(* Logix 5000 AddOnInstructionDefinition export MRSE_Yaskawa; software revision 17.00 *)

TYPE Yaskawa_EIP_Servo :   // Yaskawa SigmaLogic Axis Structure v2.4.0
STRUCT
   O : Yaskawa_OUT_to_Servo;
   I : Yaskawa_IN_from_Servo;
   AOI_SB : Yaskawa_AOI_Status_Bits;
END_STRUCT
END_TYPE

TYPE Yaskawa_OUT_to_Servo :   // Structure of data sent out to the Yaskawa SigmaLogic controller v2.4.0
STRUCT
   b00_ServoOn : BOOL;   // Servo On
   b01_Stop : BOOL;   // Stops All Current Motion in Progress
   b02_Home : BOOL;   // Start Homing Process
   b03_MoveStart1 : BOOL;   // Start Current Motion
   b06_SuperImpose : BOOL;
   b07_ServoAlarmReset : BOOL;   // Servo Alarm Reset
   b08_ControllerAlarmReset : BOOL;   // SigmaLogic Alarm Reset
   b09_MoveStart2 : BOOL;   // Start Second Motion (Blended Move)
   b10_MoveAbort : BOOL;   // Abort Current Move
   b11_MovePause : BOOL;   // Pause Current Move
   b12_SeqPause : BOOL;   // Indexing Sequence Pause
   b13_SeqResume : BOOL;   // Indexing Sequence Resume
   b14_SeqCancel : BOOL;   // Indexing Sequence Cancel
   b15_AbsEncoderReset : BOOL;   // Absolute Encoder Reset
   b16_SeqStart : BOOL;   // Start Indexing Sequence
   b17_SeqEditSpeed : BOOL;   // Enter Edit Speed
   b18_SeqEditDistance : BOOL;   // Enter Distance Edit
   b19_PLSEnable : BOOL;   // Enable PLS execution
   b20_PLSActivateOutput1 : BOOL;   // Activate PLS output1 switch logic
   b21_PLSActivateOutput2 : BOOL;   // Activate PLS output2 switch logic
   b22_PLSActivateOutput3 : BOOL;   // Activate PLS output3 switch logic
   b23_PLSActivateOutput4 : BOOL;   // Activate PLS output4 switch logic
   b24_SetClock : BOOL;   // Set the remote controller clock with data provided by the PLC
   RebootController : BOOL;
   UseExternalEncoder : BOOL;   // Use External Encoder when executing MAHSP_Yaskawa
   b32_HeatbeatAnswer : BOOL;   // Heartbeat Answer
   BrakeBypassRequest : BOOL;
   SetFwdTorqueLimit : BOOL;
   SetRevTorqueLimit : BOOL;
   TorqueLimit : DINT;
   TorqueRamp : DINT;
   HomeMethod : INT;
   HomeSpeed : DINT;
   HomeAccDec : DINT;   // Home Move Acceleration/Deceleration Rate
   HomeBackOffDistance : DINT;
   HomeCreepSpeed : DINT;
   HomeCreepDistanceLimit : DINT;
   HomeCreepTimeLimit : DINT;
   HomeOffsetDistance : DINT;
   HomeOffsetSpeed : DINT;
   HomePostion : DINT;
   HomeTorque : DINT;
   HomeInputNo : DINT;
   HomeApproachTimeLimit : DINT;
   HomeApproachDistLimit : DINT;
   HomeDirection : INT;
   HomeSwitchMode : INT;
   MoveType : INT;
   MoveDirection : INT;
   MoveAccel1 : DINT;
   MoveAccel2 : DINT;
   MoveDecel1 : DINT;
   MoveDecel2 : DINT;
   MoveSpeed1 : DINT;
   MoveSpeed2 : DINT;
   MoveDistance1 : DINT;
   MoveDistance2 : DINT;
   MovePosition1 : DINT;
   MovePosition2 : DINT;
   RegistrationDistance : DINT;
   GearNumerator : DINT;
   GearDenominator : DINT;
   SuperImposeDistance : DINT;
   Resolution : INT;
   RegistrationDirection : INT;
   TuningLevel : INT;
   SequenceStep : INT;   // Staring Sequence Step Number
   SequenceEditStep : INT;   // Sequence Step Number to Edit
   FlagCommandBits1 : DINT;   // Flag Commands. 1..64 are General Flags, Bits 0..31 correspond to Flag 1..32
   FlagCommandBits2 : DINT;   // Flag Commands cont. 1..64 are General Flags, Bits 0..31 correspond to Flag 33..64
   DigitalOutCommandBits : DINT;   // Digital Output commands. Bits 0-7 correspond to CN13 Digital Outputs 0-7, used as Flag 73-80. Bits 8-10 correspond to CN1 Digital Outputs 0-2 used as Flag 88-90"
   SequenceEditSpeed : DINT;
   SequenceEditDistance : DINT;
   FeedRateOverride : INT;
   HSI_Enable : BOOL;
   HSI_MoveMode : BOOL;   // 0=Relative; 1=Moves per Cycle
   HSI_CalcMethod : BOOL;   // 0=Accel/Decel; 1=Time
   HSI_MoveDirection : BOOL;   // 0 = Negative; 1 = Positive
   HSI_TriggerFlag : INT;
   HSI_MovingFlag : INT;
   HSI_DwellingFlag : INT;
   HSI_DoneFlag : INT;
   HSI_MoveType : INT;   // 0=Single; 1=Repeat; 2=Repeat "x" times
   HSI_RepeatNumber : INT;
   HSI_Distance : DINT;
   HSI_Speed : DINT;
   HSI_Accel : DINT;
   HSI_MoveTime : DINT;
   HSI_DwellTime : DINT;
   PLS_OutputFlag1 : INT;
   PLS_OutputFlag2 : INT;
   PLS_OutputFlag3 : INT;
   PLS_OutputFlag4 : INT;
   PLS_OnPosition1 : DINT;
   PLS_OffPosition1 : DINT;
   PLS_OnPosition2 : DINT;
   PLS_OffPosition2 : DINT;
   PLS_OnPosition3 : DINT;
   PLS_OffPosition3 : DINT;
   PLS_OnPosition4 : DINT;
   PLS_OffPosition4 : DINT;
   PLS_OnCompensation1 : INT;
   PLS_OffCompensation1 : INT;
   PLS_OnCompensation2 : INT;
   PLS_OffCompensation2 : INT;
   PLS_OnCompensation3 : INT;
   PLS_OffCompensation3 : INT;
   PLS_OnCompensation4 : INT;
   PLS_OffCompensation4 : INT;
   RTC_Year : INT;
   RTC_Month : INT;
   RTC_Day : INT;
   RTC_Hour : INT;
   RTC_Min : INT;
   RTC_Sec : INT;
   StopDecel : DINT;
   AnalogOutput : INT;   // CN13, AO_01 [mV]
END_STRUCT
END_TYPE

TYPE Yaskawa_AOI_Status_Bits :   // Internal bits used to interlock Yaskawa AOI execution. v2.4.0
STRUCT
   MAM : BOOL;   // Move AOI Active
   MAJ : BOOL;   // Jog AOI Active
   MAB : BOOL;   // Blending AOI Active
   MAG : BOOL;   // Gearing AOI Active
   MAHSP : BOOL;   // Home SetPoint AOI Active
   MAH : BOOL;   // Homing AOI Active
   MSQE : BOOL;   // Sequence Edit AOI Active
   MSQR : BOOL;   // Sequence Run AOI Active
   MHSI : BOOL;   // High Speed Index AOI Active
   MSO : BOOL;   // Servo On
   MSF : BOOL;   // Servo Off
   MAFR : BOOL;   // Fault Reset
   MAS : BOOL;   // Servo Abort
   MTRQ : BOOL;   // Torque Mode Active
   MPLS : BOOL;   // PLS Active
   MCLK : BOOL;   // SetClock Active
   MSTL : BOOL;   // Set Torque Limit Active
   AOI_Permissive : BOOL;   // Permissive to Execute an AOI
END_STRUCT
END_TYPE

TYPE Yaskawa_IN_from_Servo :   // Structure of data coming from the Yaskawa SigmaLogic controller. v2.4.0
STRUCT
   AlarmText : STRING;   // ServoPack Alarm Code plus Text Description
   b00_Heartbeat : BOOL;
   b01_Alarm : BOOL;   // ServoPack Alarm
   b02_Warning : BOOL;   // ServoPack Warning
   b03_Ready : BOOL;   // ServoPack Ready
   b04_Enabled : BOOL;   // ServoPack Enabled ("Servo On")
   b05_StopComplete : BOOL;
   b06_HomeComplete : BOOL;
   b07_HomeBusy : BOOL;
   b08_HomeActive : BOOL;
   b09_HomeAborted : BOOL;
   b10_HomeError : BOOL;
   b11_MoveAbsComplete : BOOL;
   b12_MoveAbsBusy : BOOL;
   b13_MoveAbsActive : BOOL;
   b14_MoveAbsAborted : BOOL;
   b15_MoveAbsError : BOOL;
   b16_MoveRelComplete : BOOL;
   b17_MoveRelBusy : BOOL;
   b18_MoveRelActive : BOOL;
   b19_MoveRelAborted : BOOL;
   b20_MoveRelError : BOOL;
   b21_JogAtSpeed : BOOL;
   b22_JogBusy : BOOL;
   b23_JogActive : BOOL;
   b24_JogAborted : BOOL;
   b25_JogError : BOOL;
   b26_GearInSync : BOOL;
   b27_GearBusy : BOOL;
   b28_GearActive : BOOL;
   b29_GearAborted : BOOL;
   b30_GearError : BOOL;
   b32_MoveSuperComplete : BOOL;
   b33_MoveSuperBusy : BOOL;
   b34_MoveSuperActive : BOOL;
   b35_MoveSuperAborted : BOOL;
   b36_MoveSuperError : BOOL;
   b37_PowerCycleRequired : BOOL;
   b38_MoveBlend1Complete : BOOL;
   b39_MoveBlend1Busy : BOOL;
   b40_MoveBlend1Active : BOOL;
   b41_MoveBlend1Abort : BOOL;
   b42_MoveBlend1Error : BOOL;
   b43_MoveBlend2Complete : BOOL;
   b44_MoveBlend2Busy : BOOL;
   b45_MoveBlend2Active : BOOL;
   b46_MoveBlend2Abort : BOOL;
   b47_MoveBlend2Error : BOOL;
   b48_RegComplete : BOOL;
   b49_RegBusy : BOOL;
   b50_RegActive : BOOL;
   b51_RegAborted : BOOL;
   b52_RegError : BOOL;
   b53_ResetAbsEncoderActive : BOOL;
   b54_ResetAbsEncoderBusy : BOOL;
   b55_ResetAbsEncoderDone : BOOL;
   b56_ResetAbsEncoderError : BOOL;
   b57_SeqRunning : BOOL;
   b58_RegSensorNotReached : BOOL;
   b59_SeqEditError : BOOL;
   b60_SeqEditDone : BOOL;
   b61_TorqueAtTorque : BOOL;
   b62_TorqueBusy : BOOL;
   b63_TorqueActive : BOOL;
   b64_TorqueAborted : BOOL;
   b65_TorqueError : BOOL;
   b66_ControllerAlarm : BOOL;
   b67_ApplicationError : BOOL;
   b68_AxisAtStandStill : BOOL;
   b69_TestModeActive : BOOL;
   b70_ServoParamsOK : BOOL;
   b71_SetFwdTorqueLimitDone : BOOL;
   b72_SetRevTorqueLimitDone : BOOL;
   Position : DINT;
   Speed : DINT;
   Torque : DINT;
   HomeErrorID : INT;
   MoveAbsErrorID : INT;
   MoveRelErrorID : INT;
   JogErrorID : INT;
   GearErrorID : INT;
   MoveSuperErrorID : INT;
   ServoAlarmID : INT;
   ServoWarningID : INT;
   ControllerAlarmID : DINT;
   AxisGenAlarmID : DINT;
   MoveBlend1ErrorID : INT;
   MoveBlend2ErrorID : INT;
   ResetAbsEncoderErrorID : INT;
   FunctionBlockErrorID : INT;
   TorqueErrorID : INT;
   RegErrorID : INT;
   SeqCurrentStep : INT;
   FlagStatusBit1 : DINT;   // Flag Status. 1..64 are General Flags, Bits 0..31 correspond to Flag 1..32
   FlagStatusBit2 : DINT;   // Flag Status cont. 1..64 are General Flags, Bits 0..31 correspond to Flag 33..64
   IOStatusBits : DINT;   // Digital IO Status. Bits 0-7, CN13 Inputs 0-7, Used as Flag 65-72. Bits 8-15, CN13 Outputs 0-7, Used as Flag 73-80. Bits 16-22, CN1 Inputs 0-6, Used as Flag 81-87. Bits 23-25, CN1 Outputs 0-4, Used as Flag 88-92.
   HSI_Moving : BOOL;
   HSI_Dwelling : BOOL;
   HSI_Done : BOOL;
   HSI_Busy : BOOL;
   HSI_Error : BOOL;
   HSI_ErrorCode : INT;
   PLS_Running : BOOL;
   PLS_SwitchStatus1 : BOOL;
   PLS_SwitchStatus2 : BOOL;
   PLS_SwitchStatus3 : BOOL;
   PLS_SwitchStatus4 : BOOL;
   PLS_Busy : BOOL;
   PLS_Error : BOOL;
   PLS_ErrorCode : INT;
   SetClock_Done : BOOL;
   SetClock_Busy : BOOL;
   SetClock_Error : BOOL;
   SetClock_ErrorID : INT;
   SoftwareVersion : DINT;
   FirmwareVersion : DINT;
   CommandedPos : DINT;
   CommandedPosNonCyc : DINT;
   CommandedSpeed : DINT;
   Clock_Year : INT;
   Clock_Month : INT;
   Clock_Day : INT;
   Clock_Hour : INT;
   Clock_Minute : INT;
   Clock_Second : INT;
   AnalogInput : REAL;   // CN13, AI_01 [v]
   BrakeBypassActive : BOOL;
   ForwardTorqueLimit : DINT;
   ReverseTorqueLimit : DINT;
END_STRUCT
END_TYPE

ADD_ON_INSTRUCTION MRSE_Yaskawa   (* revision 2.4 0, ExecuteEnableInFalse *)
// Motion Report Servo Error
// Alarm text will be reported to controller tag at "AxisRef.I.AlarmText"
// Revision note:
// 2.4.0: No functional change
// 2.3.1: No functional change
// 2.3.0: No functional change
// 2.0.0: First release
VAR_INPUT
   AOI_ON_LOCAL : BOOL;
END_VAR
VAR_IN_OUT
   Axis_IN : AB:ETHERNET_MODULE_DINT_256Bytes:I:0; {required}
   Axis : Yaskawa_EIP_Servo; {required}
END_VAR
VAR_OUTPUT
   EN : BOOL; {visible}   // Function is executing
   DN : BOOL; {visible}   // MRSE completed successfully
END_VAR
VAR
   OS1 : BOOL;
   OS2 : BOOL;
END_VAR

ROUTINE EnableInFalse   (* ladder *)
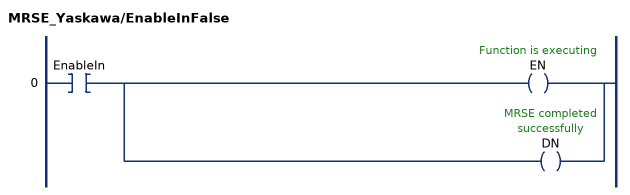
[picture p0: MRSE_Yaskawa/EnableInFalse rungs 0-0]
   0: XIC(EnableIn)[OTE(EN) ,OTE(DN) ];
END_ROUTINE

ROUTINE Logic   (* ladder *)
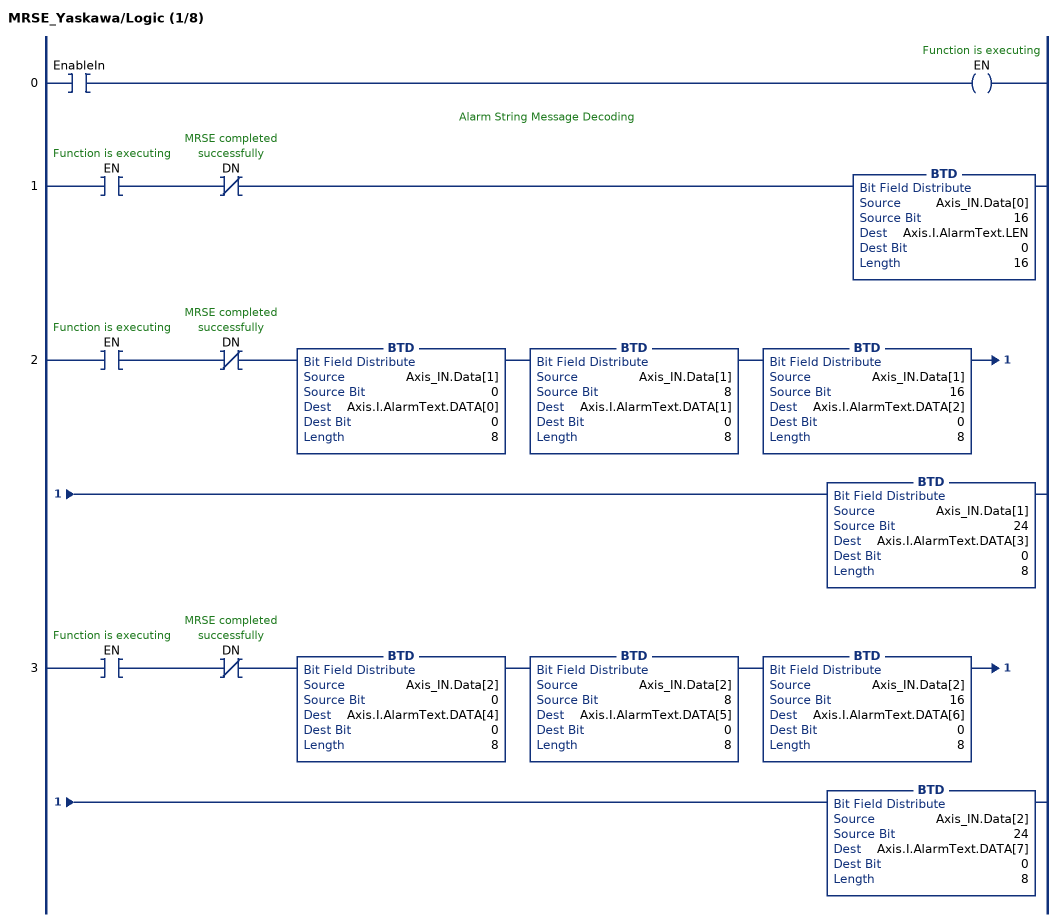
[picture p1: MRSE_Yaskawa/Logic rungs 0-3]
   0: XIC(EnableIn)OTE(EN);
   // Alarm String Message Decoding
   1: XIC(EN)XIO(DN)BTD(Axis_IN.Data[0],16,Axis.I.AlarmText.LEN,0,16);
   2: XIC(EN)XIO(DN)BTD(Axis_IN.Data[1],0,Axis.I.AlarmText.DATA[0],0,8)BTD(Axis_IN.Data[1],8,Axis.I.AlarmText.DATA[1],0,8)BTD(Axis_IN.Data[1],16,Axis.I.AlarmText.DATA[2],0,8)BTD(Axis_IN.Data[1],24,Axis.I.AlarmText.DATA[3],0,8);
   3: XIC(EN)XIO(DN)BTD(Axis_IN.Data[2],0,Axis.I.AlarmText.DATA[4],0,8)BTD(Axis_IN.Data[2],8,Axis.I.AlarmText.DATA[5],0,8)BTD(Axis_IN.Data[2],16,Axis.I.AlarmText.DATA[6],0,8)BTD(Axis_IN.Data[2],24,Axis.I.AlarmText.DATA[7],0,8);
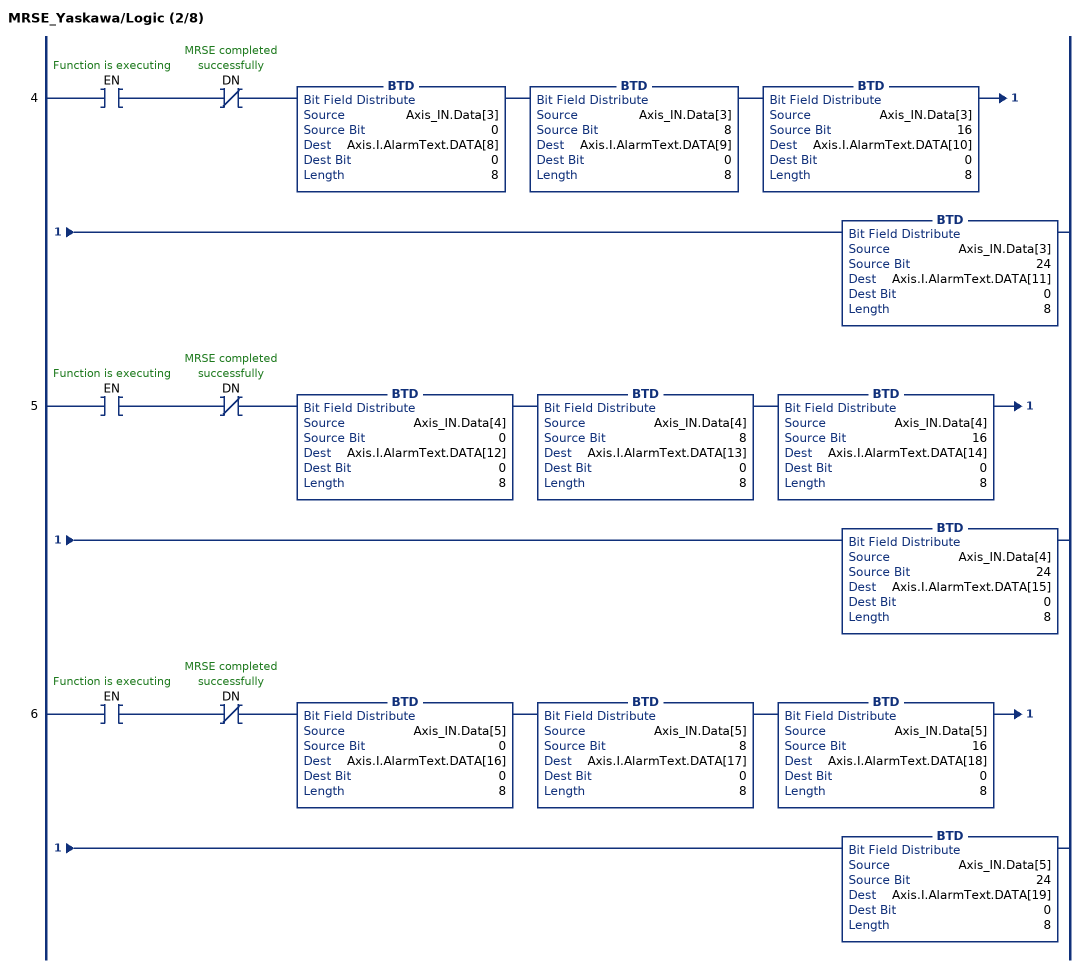
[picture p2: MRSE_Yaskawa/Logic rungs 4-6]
   4: XIC(EN)XIO(DN)BTD(Axis_IN.Data[3],0,Axis.I.AlarmText.DATA[8],0,8)BTD(Axis_IN.Data[3],8,Axis.I.AlarmText.DATA[9],0,8)BTD(Axis_IN.Data[3],16,Axis.I.AlarmText.DATA[10],0,8)BTD(Axis_IN.Data[3],24,Axis.I.AlarmText.DATA[11],0,8);
   5: XIC(EN)XIO(DN)BTD(Axis_IN.Data[4],0,Axis.I.AlarmText.DATA[12],0,8)BTD(Axis_IN.Data[4],8,Axis.I.AlarmText.DATA[13],0,8)BTD(Axis_IN.Data[4],16,Axis.I.AlarmText.DATA[14],0,8)BTD(Axis_IN.Data[4],24,Axis.I.AlarmText.DATA[15],0,8);
   6: XIC(EN)XIO(DN)BTD(Axis_IN.Data[5],0,Axis.I.AlarmText.DATA[16],0,8)BTD(Axis_IN.Data[5],8,Axis.I.AlarmText.DATA[17],0,8)BTD(Axis_IN.Data[5],16,Axis.I.AlarmText.DATA[18],0,8)BTD(Axis_IN.Data[5],24,Axis.I.AlarmText.DATA[19],0,8);
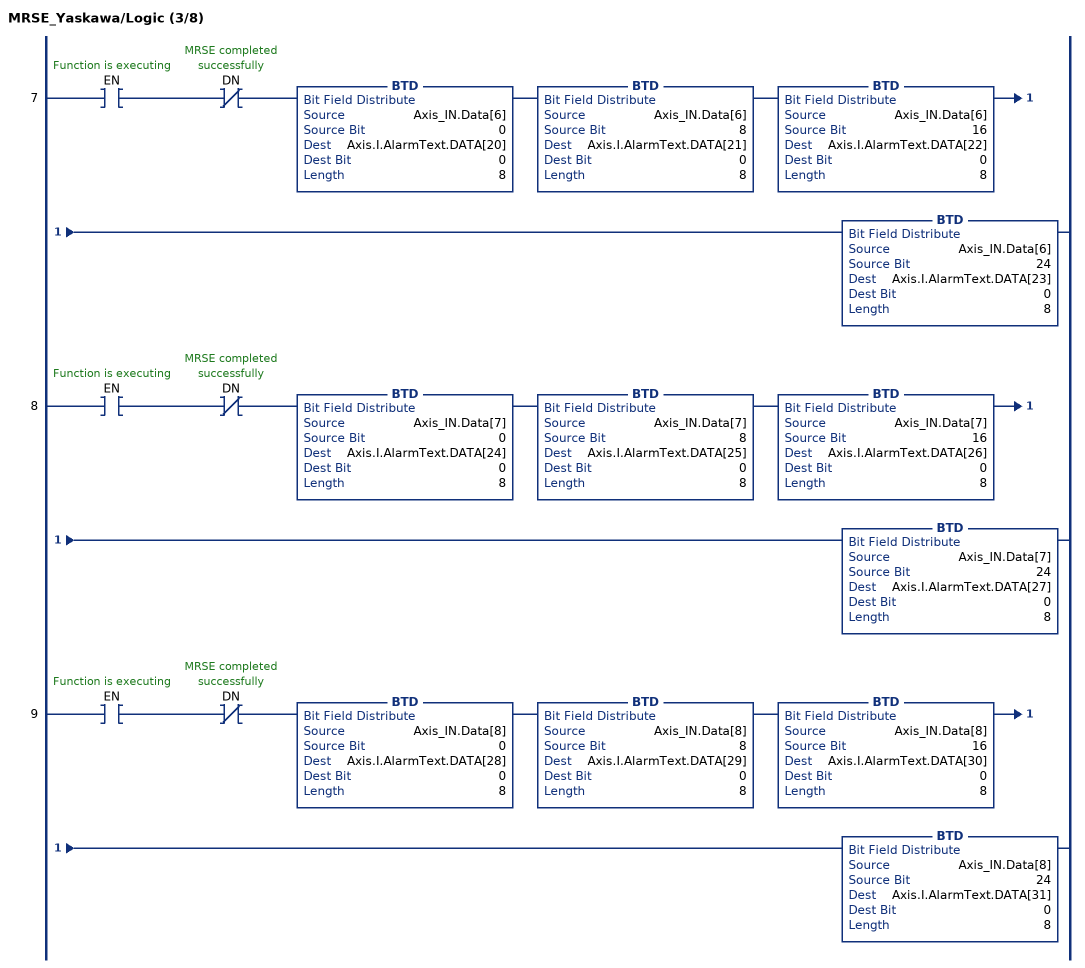
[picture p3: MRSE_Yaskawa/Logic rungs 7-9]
   7: XIC(EN)XIO(DN)BTD(Axis_IN.Data[6],0,Axis.I.AlarmText.DATA[20],0,8)BTD(Axis_IN.Data[6],8,Axis.I.AlarmText.DATA[21],0,8)BTD(Axis_IN.Data[6],16,Axis.I.AlarmText.DATA[22],0,8)BTD(Axis_IN.Data[6],24,Axis.I.AlarmText.DATA[23],0,8);
   8: XIC(EN)XIO(DN)BTD(Axis_IN.Data[7],0,Axis.I.AlarmText.DATA[24],0,8)BTD(Axis_IN.Data[7],8,Axis.I.AlarmText.DATA[25],0,8)BTD(Axis_IN.Data[7],16,Axis.I.AlarmText.DATA[26],0,8)BTD(Axis_IN.Data[7],24,Axis.I.AlarmText.DATA[27],0,8);
   9: XIC(EN)XIO(DN)BTD(Axis_IN.Data[8],0,Axis.I.AlarmText.DATA[28],0,8)BTD(Axis_IN.Data[8],8,Axis.I.AlarmText.DATA[29],0,8)BTD(Axis_IN.Data[8],16,Axis.I.AlarmText.DATA[30],0,8)BTD(Axis_IN.Data[8],24,Axis.I.AlarmText.DATA[31],0,8);
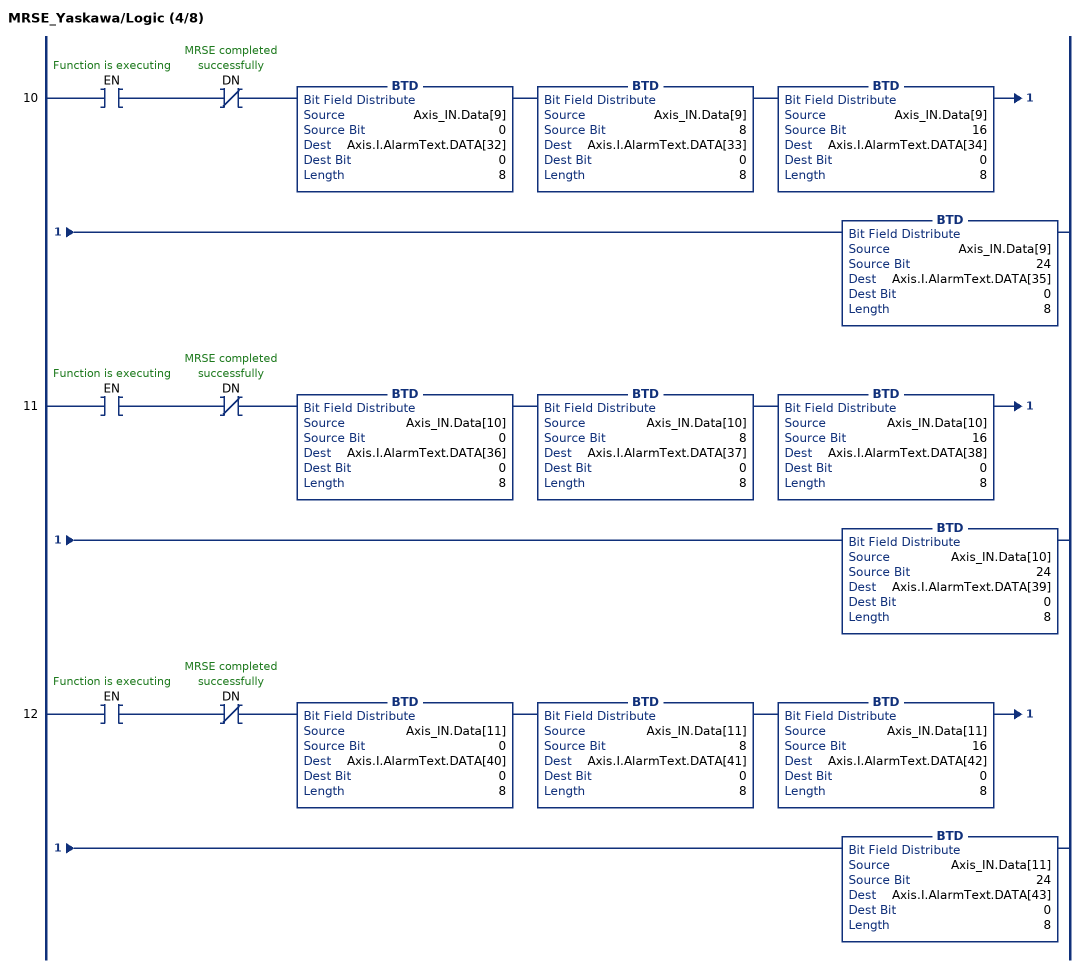
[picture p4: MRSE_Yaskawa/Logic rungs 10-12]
   10: XIC(EN)XIO(DN)BTD(Axis_IN.Data[9],0,Axis.I.AlarmText.DATA[32],0,8)BTD(Axis_IN.Data[9],8,Axis.I.AlarmText.DATA[33],0,8)BTD(Axis_IN.Data[9],16,Axis.I.AlarmText.DATA[34],0,8)BTD(Axis_IN.Data[9],24,Axis.I.AlarmText.DATA[35],0,8);
   11: XIC(EN)XIO(DN)BTD(Axis_IN.Data[10],0,Axis.I.AlarmText.DATA[36],0,8)BTD(Axis_IN.Data[10],8,Axis.I.AlarmText.DATA[37],0,8)BTD(Axis_IN.Data[10],16,Axis.I.AlarmText.DATA[38],0,8)BTD(Axis_IN.Data[10],24,Axis.I.AlarmText.DATA[39],0,8);
   12: XIC(EN)XIO(DN)BTD(Axis_IN.Data[11],0,Axis.I.AlarmText.DATA[40],0,8)BTD(Axis_IN.Data[11],8,Axis.I.AlarmText.DATA[41],0,8)BTD(Axis_IN.Data[11],16,Axis.I.AlarmText.DATA[42],0,8)BTD(Axis_IN.Data[11],24,Axis.I.AlarmText.DATA[43],0,8);
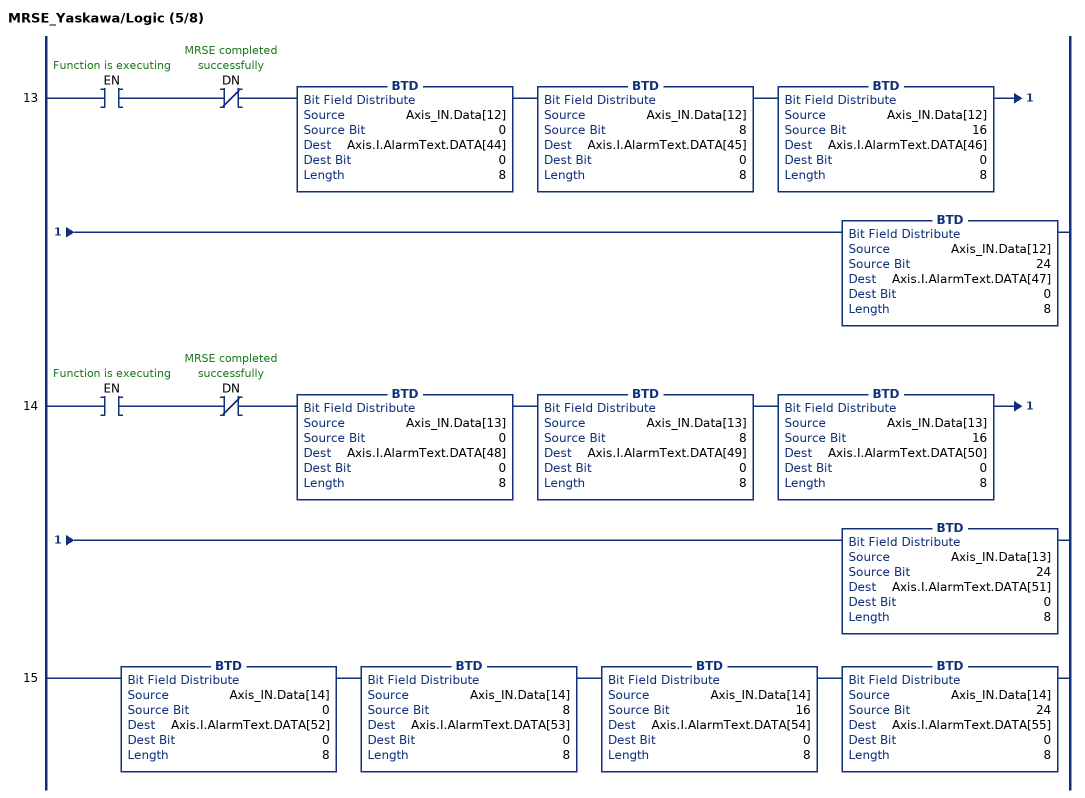
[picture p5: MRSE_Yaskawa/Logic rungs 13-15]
   13: XIC(EN)XIO(DN)BTD(Axis_IN.Data[12],0,Axis.I.AlarmText.DATA[44],0,8)BTD(Axis_IN.Data[12],8,Axis.I.AlarmText.DATA[45],0,8)BTD(Axis_IN.Data[12],16,Axis.I.AlarmText.DATA[46],0,8)BTD(Axis_IN.Data[12],24,Axis.I.AlarmText.DATA[47],0,8);
   14: XIC(EN)XIO(DN)BTD(Axis_IN.Data[13],0,Axis.I.AlarmText.DATA[48],0,8)BTD(Axis_IN.Data[13],8,Axis.I.AlarmText.DATA[49],0,8)BTD(Axis_IN.Data[13],16,Axis.I.AlarmText.DATA[50],0,8)BTD(Axis_IN.Data[13],24,Axis.I.AlarmText.DATA[51],0,8);
   15: BTD(Axis_IN.Data[14],0,Axis.I.AlarmText.DATA[52],0,8)BTD(Axis_IN.Data[14],8,Axis.I.AlarmText.DATA[53],0,8)BTD(Axis_IN.Data[14],16,Axis.I.AlarmText.DATA[54],0,8)BTD(Axis_IN.Data[14],24,Axis.I.AlarmText.DATA[55],0,8);
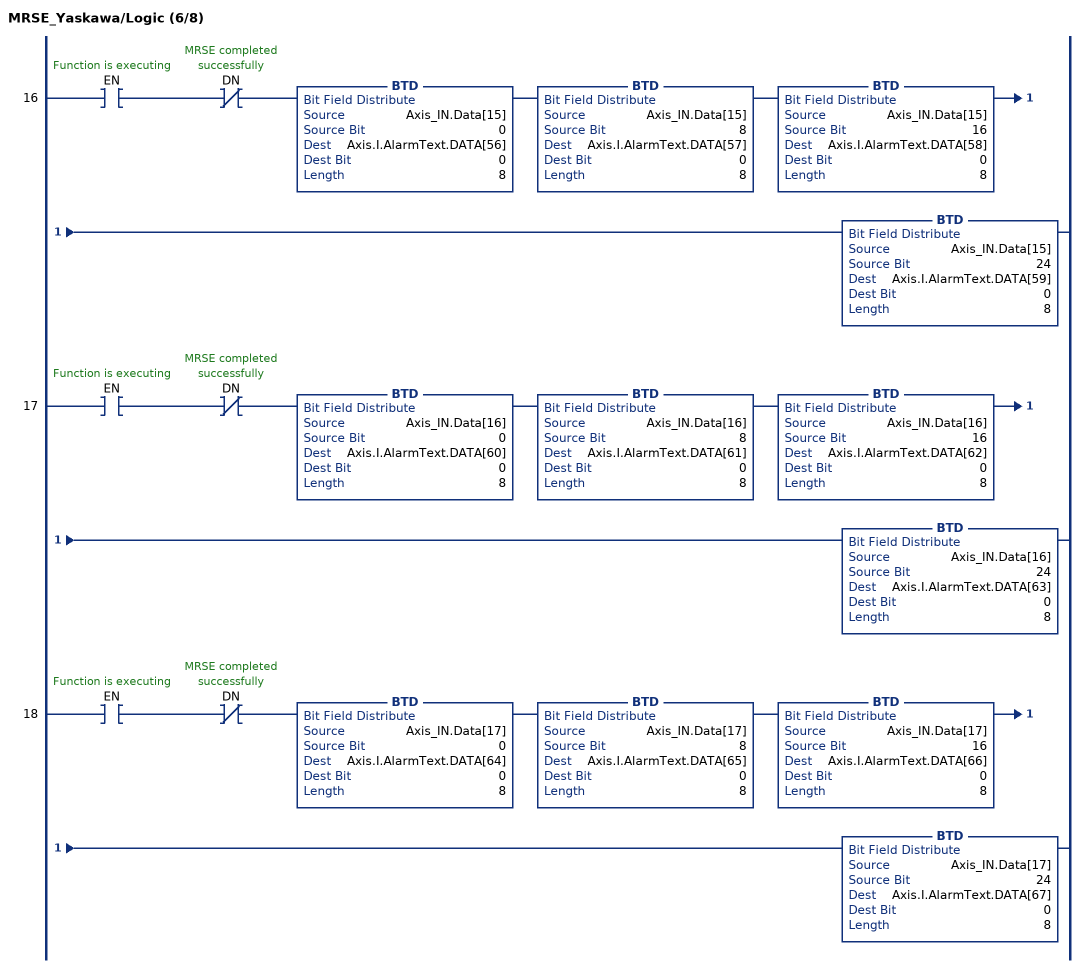
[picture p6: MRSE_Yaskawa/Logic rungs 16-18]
   16: XIC(EN)XIO(DN)BTD(Axis_IN.Data[15],0,Axis.I.AlarmText.DATA[56],0,8)BTD(Axis_IN.Data[15],8,Axis.I.AlarmText.DATA[57],0,8)BTD(Axis_IN.Data[15],16,Axis.I.AlarmText.DATA[58],0,8)BTD(Axis_IN.Data[15],24,Axis.I.AlarmText.DATA[59],0,8);
   17: XIC(EN)XIO(DN)BTD(Axis_IN.Data[16],0,Axis.I.AlarmText.DATA[60],0,8)BTD(Axis_IN.Data[16],8,Axis.I.AlarmText.DATA[61],0,8)BTD(Axis_IN.Data[16],16,Axis.I.AlarmText.DATA[62],0,8)BTD(Axis_IN.Data[16],24,Axis.I.AlarmText.DATA[63],0,8);
   18: XIC(EN)XIO(DN)BTD(Axis_IN.Data[17],0,Axis.I.AlarmText.DATA[64],0,8)BTD(Axis_IN.Data[17],8,Axis.I.AlarmText.DATA[65],0,8)BTD(Axis_IN.Data[17],16,Axis.I.AlarmText.DATA[66],0,8)BTD(Axis_IN.Data[17],24,Axis.I.AlarmText.DATA[67],0,8);
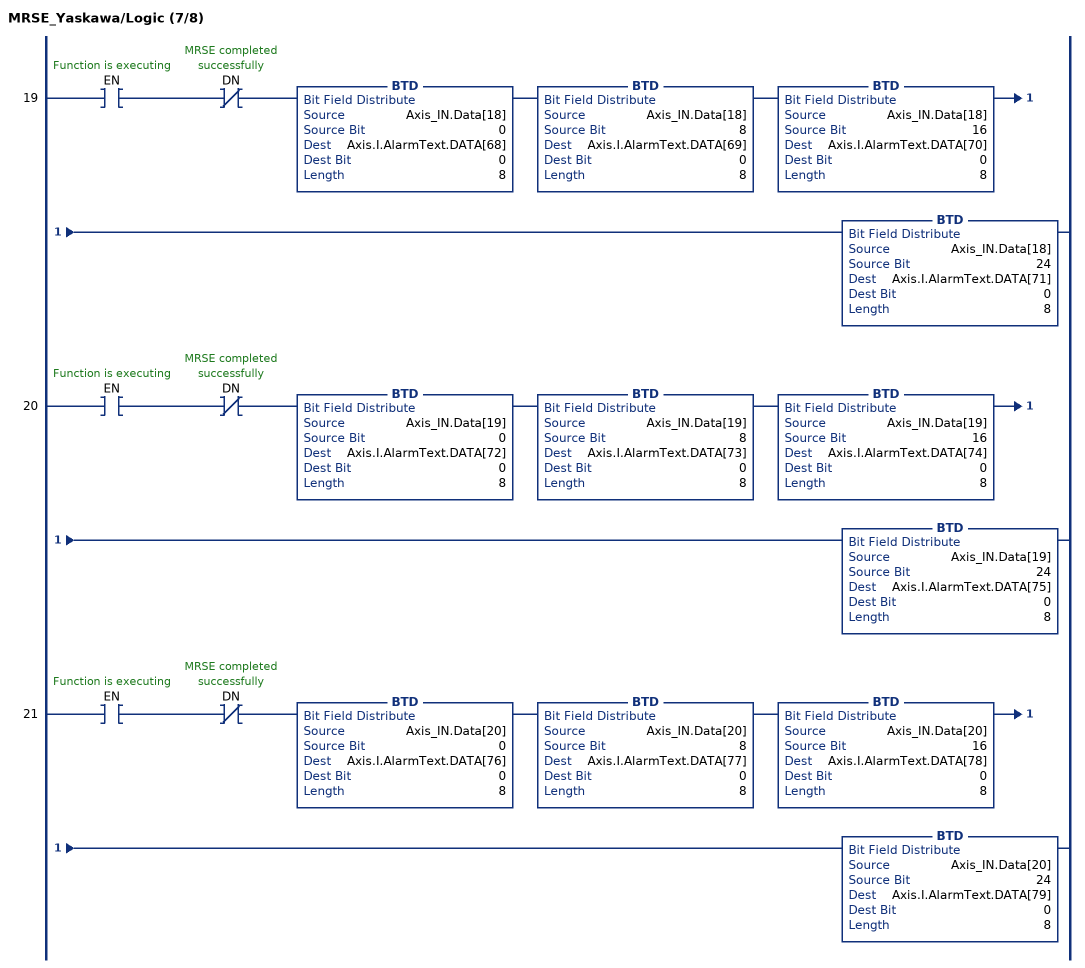
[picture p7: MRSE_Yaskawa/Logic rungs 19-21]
   19: XIC(EN)XIO(DN)BTD(Axis_IN.Data[18],0,Axis.I.AlarmText.DATA[68],0,8)BTD(Axis_IN.Data[18],8,Axis.I.AlarmText.DATA[69],0,8)BTD(Axis_IN.Data[18],16,Axis.I.AlarmText.DATA[70],0,8)BTD(Axis_IN.Data[18],24,Axis.I.AlarmText.DATA[71],0,8);
   20: XIC(EN)XIO(DN)BTD(Axis_IN.Data[19],0,Axis.I.AlarmText.DATA[72],0,8)BTD(Axis_IN.Data[19],8,Axis.I.AlarmText.DATA[73],0,8)BTD(Axis_IN.Data[19],16,Axis.I.AlarmText.DATA[74],0,8)BTD(Axis_IN.Data[19],24,Axis.I.AlarmText.DATA[75],0,8);
   21: XIC(EN)XIO(DN)BTD(Axis_IN.Data[20],0,Axis.I.AlarmText.DATA[76],0,8)BTD(Axis_IN.Data[20],8,Axis.I.AlarmText.DATA[77],0,8)BTD(Axis_IN.Data[20],16,Axis.I.AlarmText.DATA[78],0,8)BTD(Axis_IN.Data[20],24,Axis.I.AlarmText.DATA[79],0,8);
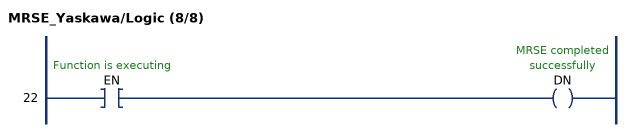
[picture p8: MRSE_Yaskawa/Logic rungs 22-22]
   22: XIC(EN)OTE(DN);
END_ROUTINE
END_ADD_ON_INSTRUCTION
